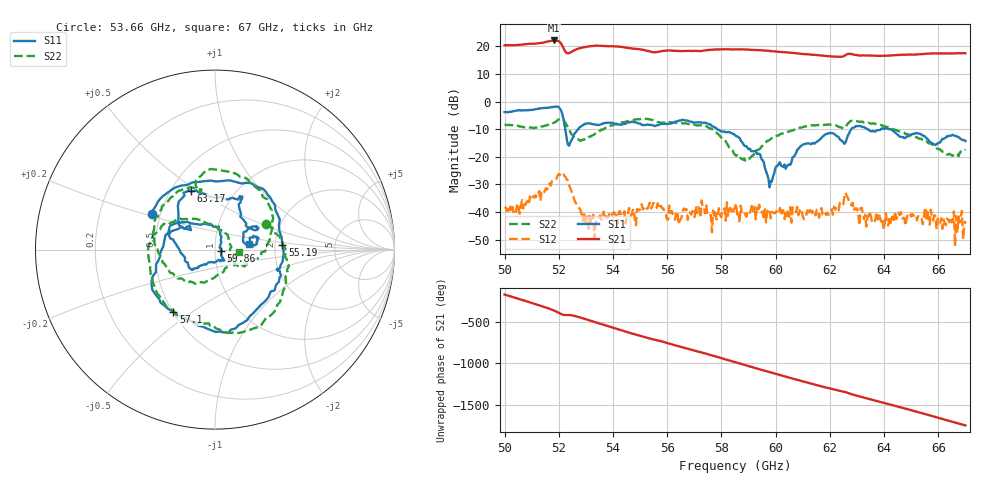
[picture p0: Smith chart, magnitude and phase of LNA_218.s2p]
!Agilent Technologies,E8361A,US42410132,A.06.03.05
!Agilent E8361A: A.06.03.05
!Date: Friday, July 11, 2008 12:48:42
!Correction: S11(Full 2 Port(1,2)) S21(Full 2 Port(1,2)) S12(Full 2 Port(1,2)) S22(Full 2 Port(1,2))
!S2P File: Measurements: S11, S21, S12, S22:
# Hz S  MA  R 50
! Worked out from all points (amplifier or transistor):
!   401 points, 50 GHz to 67 GHz, reference 50 ohm
!   highest |S21| = 22.2 dB at 51.83 GHz (marker M1)
!   |S21| within 3 dB of that: start of sweep to 52.18 GHz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
!   unconditionally stable (mu >= 1): start of sweep to 50.92 GHz; 50.96751 GHz to 51.02164 GHz; 52.22 GHz to end of sweep
!   at 52.8 GHz: K = 4.19, MAG = 20.2 dB, |S12| = -39.3 dB
!   at 58.5 GHz: K = 4.49, MAG = 19.2 dB, |S12| = -38.5 dB
!   at 67 GHz: K = 9.14, MAG = 17.8 dB, |S12| = -43.2 dB
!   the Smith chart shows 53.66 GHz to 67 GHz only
!   S11 on the Smith chart (normalised r, x): 53.66 GHz: 0.45, +0.21; 55.19 GHz: 2.19, +0.14; 57.1 GHz: 0.50, -0.42; 59.86 GHz: 1.07, -0.02; 63.17 GHz: 0.63, +0.47; 67 GHz: 1.47, +0.10
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5e10  0.6468 118.2  10.49 -169.1  0.01226 -31.6  0.384 25.3
5.09775e10  0.707 26.6  11.22 91.6  0.01671 -117.8  0.3412 -46.0
5.18275e10  0.8056 -63.7  12.81 -3.4  0.03918 155.3  0.4161 -136.6
5.20825e10  0.6919 -114.9  11.3 -44.2  0.05108 98.7  0.4877 159.7
5.28475e10  0.3634 -123.1  9.52 -92.6  0.008614 -19.7  0.2023 70.8
5.3655e10  0.4042 150.8  10.19 -176.6  0.01015 -26.6  0.3158 26.4
5.442e10  0.3948 72.2  9.602 106.1  0.01032 -69.0  0.42 -21.0
5.5185e10  0.3762 4.2  8.505 33.4  0.0128 -118.5  0.4879 -66.2
5.5695e10  0.3813 -18.6  8.008 -7.1  0.01153 156.6  0.4249 -93.7
5.6375e10  0.4407 -72.9  8.275 -70.9  0.01003 124.3  0.4126 -125.9
5.70975e10  0.4181 -123.7  8.234 -135.9  0.009588 82.1  0.3704 -166.7
5.77775e10  0.3383 -166.0  8.84 162.7  0.01025 3.4  0.2759 145.6
5.85e10  0.2473 143.5  8.839 93.3  0.01191 -58.6  0.109 75.9
5.92225e10  0.1261 82.6  8.624 24.2  0.01239 -69.9  0.1188 -53.5
5.986e10  0.03563 -14.0  8.182 -35.8  0.01006 -154.9  0.2193 -119.8
6.054e10  0.07166 -104.1  7.716 -98.2  0.01232 153.7  0.2916 -164.0
6.13475e10  0.1756 -157.1  7.082 -170.1  0.009601 100.7  0.3729 153.0
6.258e10  0.1824 142.4  6.98 90.1  0.02256 -5.0  0.3445 106.5
6.3175e10  0.3522 112.7  6.859 31.7  0.01193 -71.8  0.4337 67.0
6.4195e10  0.3159 62.4  6.818 -56.9  0.007842 -133.2  0.334 18.6
6.55975e10  0.2114 31.2  7.378 177.2  0.01122 111.6  0.1839 -29.6
6.7e10  0.1933 9.6  7.505 46.9  0.006888 -13.4  0.1363 -5.5
